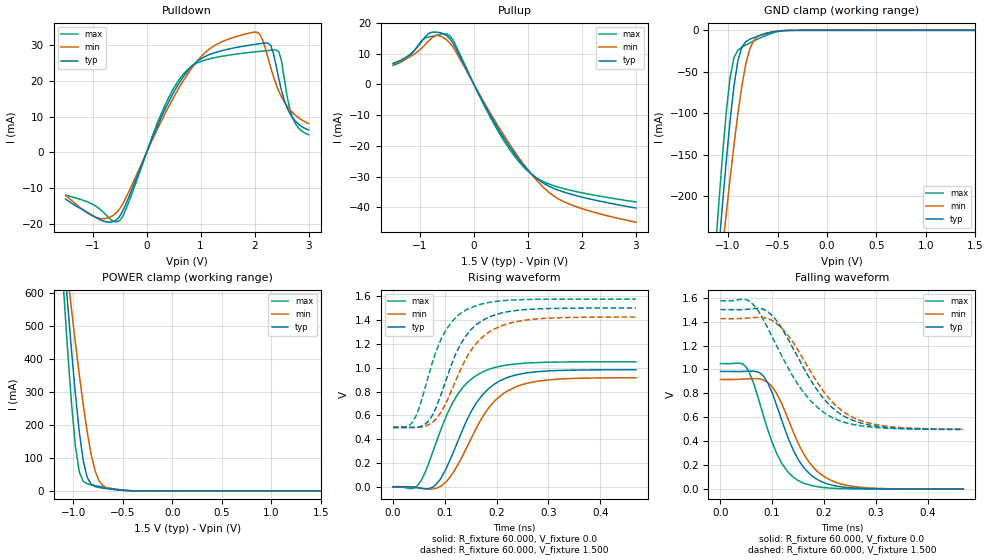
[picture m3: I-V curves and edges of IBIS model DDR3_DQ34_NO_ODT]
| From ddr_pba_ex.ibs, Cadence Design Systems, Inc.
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|   Model DDR3_DQ34_NO_ODT
[Model]   DDR3_DQ34_NO_ODT
Model_type I/O
Polarity   Non-Inverting
Enable   Active-High
Vinl   =   0.575V
Vinh   =   0.925V
C_comp   1.612pF   1.592pF   1.671pF
C_comp_pullup   0.459pF   0.494pF   0.467pF
C_comp_pulldown 1.152pF   1.097pF   1.204pF
[Model Spec]
Vinh   0.925V   NA   NA
Vinl   0.575V   NA   NA
Vmeas   0.750V   NA   NA
[Temperature Range]   27.000   0.125k   -40.000
[Voltage Range]   1.500V   1.425V   1.575V
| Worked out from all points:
|   slope of the pulldown table from 0 to 0.225 V, typ, clamps not added: 27.2 ohm
|   slope of the pullup table from 0 to 0.225 V, typ, clamps not added: 29.9 ohm
|   GND clamp passes 1 mA (typ) near -0.50 V on its own axis
|   POWER clamp passes 1 mA (typ) near -0.45 V on its own axis
|   rising waveform, R_fixture 60.000, V_fixture 0.0: 20-80 % time 68.7ps typ, 74.1ps min, 66ps max; typ from 0 V to 0.983 V
|   rising waveform, R_fixture 60.000, V_fixture 1.500: 20-80 % time 60.9ps typ, 68.7ps min, 55ps max; typ from 0.497 V to 1.5 V
|   falling waveform, R_fixture 60.000, V_fixture 0.0: 20-80 % time 56.7ps typ, 62.8ps min, 52ps max; typ from 0.983 V to 0 V
|   falling waveform, R_fixture 60.000, V_fixture 1.500: 20-80 % time 87ps typ, 87.9ps min, 89.7ps max; typ from 1.5 V to 0.498 V
[Pulldown]
|Voltage   I(typ)   I(min)   I(max)
-1.5V     -13.11mA   -12.09mA   -11.99mA
-900mV    -18.6mA    -18.43mA   -15.54mA
-500mV    -17.95mA   -15.85mA   -19.12mA
250mV     9.123mA    8.086mA    10.11mA
600mV     19.39mA    18.08mA    20.34mA
1.1V      27mA       28.19mA    25.96mA
1.7V      29.51mA    32.65mA    27.63mA
2.1V      30.49mA    33.01mA    28.32mA
2.3V      29.93mA    23.73mA    28.62mA
2.45V     20.53mA    17.11mA    28.23mA
2.7V      9.751mA    11.19mA    9.851mA
3V        6.277mA    8.093mA    4.942mA
[Pullup]
|Voltage   I(typ)   I(min)   I(max)
-1.5V     6.892mA    6.626mA    6.196mA
-1.2V     9.586mA    8.882mA    9.221mA
-950mV    14.51mA    12.17mA    14.57mA
-800mV    16.94mA    14.89mA    15.59mA
-650mV    16.95mA    15.91mA    16.25mA
-500mV    15.86mA    14.42mA    16.44mA
-350mV    12.21mA    11.08mA    13.19mA
450mV     -14.47mA   -13.63mA   -15.32mA
1V        -27.96mA   -27.83mA   -28.29mA
1.35V     -32.83mA   -34.57mA   -32.17mA
1.65V     -34.98mA   -38.1mA    -33.88mA
3V        -40.28mA   -44.89mA   -38.3mA
[GND_clamp]
|Voltage   I(typ)   I(min)   I(max)
-1.5V     -902.4mA   -795.2mA   -923mA
-1.14V    -333.6mA   -361.2mA   -285.4mA
-1.1V     -273.5mA   -314.1mA   -219.4mA
-1.06V    -215.4mA   -267.9mA   -157.1mA
-1.02V    -160.2mA   -222.9mA   -101.2mA
-980mV    -109.7mA   -179.4mA   -57.37mA
-940mV    -66.97mA   -138.2mA   -32.78mA
-900mV    -36.37mA   -100.2mA   -23.99mA
-820mV    -13.67mA   -40.29mA   -17.69mA
-740mV    -8.766mA   -12.21mA   -12.83mA
-540mV    -1.803mA   -1.643mA   -2.86mA
1.5V      1.911nA    275.5nA    464.3pA
[POWER_clamp]
|Voltage   I(typ)   I(min)   I(max)
-1.5V     2.395A     1.917A     2.689A
-1.1V     728.2mA    767.9mA    617.4mA
-1.06V    575.5mA    659.2mA    435.4mA
-1.02V    430.1mA    553.1mA    270.8mA
-980mV    295.8mA    450.4mA    137.9mA
-940mV    179.3mA    352.3mA    58.02mA
-900mV    91.53mA    260.8mA    29.3mA
-860mV    41.11mA    178.7mA    21.47mA
-780mV    13.3mA     60.49mA    15.94mA
-740mV    10.3mA     30.45mA    13.76mA
-620mV    5.486mA    5.676mA    7.71mA
1.5V      -5.523nA   -199nA     -1.165nA
[Ramp]
| variable   typ   min   max
dV/dt_r 0.549/66.986p   0.512/74.961p   0.586/65.401p
dV/dt_f 0.559/88.075p   0.516/88.502p   0.597/91.251p
R_load = 50.000
| The next line is not an IBIS keyword
| [Initial Delay]   0.225ns   0.350ns   0.175ns
[Rising Waveform]
R_fixture= 60.000
V_fixture= 0.0
V_fixture_min= 0.0
V_fixture_max= 0.0
|time   V(typ)   V(min)   V(max)
0s        462.5uV    1.599mV    3.085mV
46ps      -4.213mV   -6.217mV   6.451mV
62ps      -14.35mV   -14.98mV   121.4mV
82ps      16.7mV     -11.93mV   358.3mV
101ps     139.8mV    38.3mV     575.7mV
123ps     362.1mV    170.2mV    764.9mV
167ps     741.2mV    544.4mV    951.4mV
202ps     879.4mV    744.7mV    1.008V
250ps     950.8mV    859.3mV    1.037V
469ps     983.1mV    916.3mV    1.05V
[Rising Waveform]
R_fixture= 60.000
V_fixture= 1.500
V_fixture_min= 1.425
V_fixture_max= 1.575
|time   V(typ)   V(min)   V(max)
0s        497.3mV    500.3mV    501.9mV
38ps      498.6mV    498.6mV    545.4mV
67ps      544.5mV    519mV      911.4mV
83ps      665.6mV    568.7mV    1.136V
102ps     893.3mV    701.5mV    1.314V
121ps     1.115V     890.8mV    1.419V
143ps     1.28V      1.093V     1.489V
176ps     1.404V     1.269V     1.539V
230ps     1.475V     1.378V     1.567V
469ps     1.5V       1.425V     1.575V
[Falling Waveform]
R_fixture= 60.000
V_fixture= 0.0
V_fixture_min= 0.0
V_fixture_max= 0.0
|time   V(typ)   V(min)   V(max)
0s        983.4mV    916.2mV    1.05V
49ps      984.9mV    920.7mV    1.024V
64ps      986.9mV    923.7mV    886.6mV
83ps      944.7mV    911.5mV    615.7mV
118ps     582.1mV    719.3mV    220.2mV
141ps     322.6mV    475.2mV    100.8mV
158ps     198.7mV    315.9mV    54.87mV
188ps     79.17mV    144.7mV    20.02mV
242ps     14.8mV     33.96mV    3.478mV
469ps     191.3uV    131uV      96.01uV
[Falling Waveform]
R_fixture= 60.000
V_fixture= 1.500
V_fixture_min= 1.425
V_fixture_max= 1.575
|time   V(typ)   V(min)   V(max)
0s        1.5V       1.424V     1.574V
55ps      1.504V     1.43V      1.573V
73ps      1.512V     1.436V     1.491V
93ps      1.478V     1.423V     1.333V
128ps     1.274V     1.301V     1.034V
159ps     1.026V     1.095V     817mV
216ps     681.3mV    729.3mV    598.7mV
253ps     580.4mV    606.3mV    543.3mV
293ps     531.3mV    546.6mV    518mV
469ps     497.9mV    501.4mV    500.2mV
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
